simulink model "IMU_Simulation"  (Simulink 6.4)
settings: Solver=FixedStepDiscrete  StartTime=0.0  StopTime=25  FixedStep=.001  RelTol=1e-3
PreLoadFcn:
  | Script_Kalman
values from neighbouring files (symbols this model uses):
  Az = [1 -Ts ;0 1]    [Script_Kalman.m]
  Kz = 1e-3*[.4 ; -.04]    [Script_Kalman.m]
  Ts = .001    (= 0.001)    [Script_Kalman.m]
undefined symbols (not defined in the file or in its folder): dend, DiscIntNeverNeededParam, float, gaind, numd, polesd, tustin, zerosd
libraries: simulink x38
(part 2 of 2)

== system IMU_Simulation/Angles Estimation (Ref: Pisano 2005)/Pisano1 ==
  note: Probleme du filtrage de l'accelero : dephasage si variation rapide et de forte amplitude, fausse le calcul de l'offset Si on filtre moins, on se prend le biais du aux accelerations
  Gyro : Inport  Orientation=down
  Accel : Inport  Orientation=down  Port=2
  Adapt : Inport  Orientation=down  Port=3
  Constant : Constant  Orientation=left  Value=0  OutDataType=sfix(16)  OutScaling=2^0
  Gain6 : Gain  Orientation=left  Gain=1e-3  Multiplication=Matrix(K*u)  ParameterDataType=sfix(16)  ParameterScaling=2^0  OutDataType=sfix(16)  OutScaling=2^0
  Gain7 : Gain  Orientation=down  Gain=Ts  Multiplication=Matrix(K*u)  ParameterDataType=sfix(16)  ParameterScaling=2^0  OutDataType=sfix(16)  OutScaling=2^0
  Low Pass1 : Subsystem  Orientation=down  mask(DiscretizedZeroPole){Zeros=[], Poles=[-30*2*pi], Gain=30*2*pi, AbsTol=auto, SampleTime=.001, method=tustin, Wc=1}
      mask prompts: Zeros "Zeros (enter in s-main:)"; Poles "Poles (enter in s-domain:)"; Gain "Gain (enter in s-domain:)"; AbsTol "Absolute tolerance:"; SampleTime "Sample time:"; Wc "Critical Frequency (Hz):"
      mask help: Continuous mask uses c2d to transform parameters onto the Discrete Zero-Pole block inside.
      mask init:
      | st=SampleTime;
      | if length(st)>1
      |     st=SampleTime(1);
      | end
      | if(st>0)
      |     [zerosd,polesd,gaind] = sldiscutil('disczpk', {st,method,Wc,Zeros,Poles,Gain});
      | end	
      | s = get_param(gcb,'maskvalues');
      | zeross = s{1};
      | poless = s{2};
      | gainss = s{3};
      | %zerosc = eval(zeross);
      | %polesc = eval(poless);
      | %gainsc = eval(gainss);
      | sldiscutil('initzpkmask', st);
      | if(st==0)
      | set_param([gcb '/Zero Pole'], 'AbsoluteTolerance', AbsTol);
      | end
  Multiport Switch : MultiPortSwitch  Orientation=left  Inputs=2  zeroidx=on
  Sum2 : Sum  Inputs=++|  OutDataType=sfix(16)  OutScaling=2^0
  Sum4 : Sum  Inputs=++|  OutDataType=sfix(16)  OutScaling=2^0
  Sum5 : Sum  Orientation=left  Inputs=+-  OutDataType=sfix(16)  OutScaling=2^0
  Unit Delay2 : UnitDelay  SampleTime=-1
  Position : Outport  Orientation=up  OutDataType=sfix(16)  OutScaling=2^0
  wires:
  Sum4/1 -> Unit Delay2/1, Position/1
  Constant/1 -> Multiport Switch/2
  Gain6/1 -> Multiport Switch/3
  Adapt/1 -> Multiport Switch/1
  Multiport Switch/1 -> Sum4/1
  Sum2/1 -> Sum4/2
  Sum5/1 -> Gain6/1
  Gain7/1 -> Sum2/1
  Accel/1 -> Low Pass1/1(In1)
  Gyro/1 -> Gain7/1
  Unit Delay2/1 -> Sum5/2, Sum2/2
  Low Pass1/1(Out1) -> Sum5/1

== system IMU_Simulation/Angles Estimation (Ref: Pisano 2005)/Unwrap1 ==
  Estimated Angle : Inport
  Compare To Constant : simulink/Logic and Bit Operations/Compare To Constant  SystemSampleTime=-1  relop=>  const=180  LogicOutDataTypeMode=uint8  ZeroCross=off
  Compare To Constant1 : simulink/Logic and Bit Operations/Compare To Constant  SystemSampleTime=-1  relop=<  const=-180  LogicOutDataTypeMode=uint8  ZeroCross=off
  Compare To Zero : simulink/Logic and Bit Operations/Compare To Zero  SystemSampleTime=-1  relop=~=  LogicOutDataTypeMode=uint8  ZeroCross=off
  Difference : simulink/Discrete/Difference  SystemSampleTime=-1  ICPrevInput=0.0  OutDataType=sfix(16)  OutScaling=2^-10  DoSatur=off
  Discrete-Time Integrator : DiscreteIntegrator  gainval=1000  SampleTime=-1  OutDataType=sfix(16)  OutScaling=2^0  ICPrevOutput=DiscIntNeverNeededParam  ICPrevScaledInput=DiscIntNeverNeededParam
  Logical Operator : Logic  Orientation=up  Operator=NOR  AllPortsSameDT=off  OutDataTypeMode=boolean
  Lookup Table : Lookup  Orientation=left  InputValues=[-500 -195 195]  OutputValues=[+360 0 -360]  LookUpMeth=Use Input Below  OutDataType=sfix(16)  OutScaling=2^0
  Merge : Merge  Inputs=3
  Sum2 : Sum  OutDataType=sfix(16)  OutScaling=2^0
  unwrap : Subsystem  TreatAsAtomicUnit=on
  unwrap1 : Subsystem  TreatAsAtomicUnit=on
  unwrap2 : Subsystem  TreatAsAtomicUnit=on
  unwrap angle : Outport
  Wrap : Outport  Port=2
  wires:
  Discrete-Time Integrator/1 -> unwrap angle/1, Lookup Table/1
  Estimated Angle/1 -> Difference/1
  unwrap1/1(Out1) -> Merge/3
  unwrap/1(Out1) -> Merge/2
  unwrap2/1(Out1) -> Merge/1
  Logical Operator/1 -> unwrap2/Enable
  Compare To Constant1/1 -> Logical Operator/2, unwrap1/Enable
  Compare To Constant/1 -> unwrap/Enable, Logical Operator/1
  Difference/1 -> unwrap2/1(In1), unwrap1/1(In1), Compare To Constant1/1, unwrap/1(In1), Compare To Constant/1
  Sum2/1 -> Discrete-Time Integrator/1
  Merge/1 -> Sum2/2
  Lookup Table/1 -> Sum2/1, Compare To Zero/1
  Compare To Zero/1 -> Wrap/1

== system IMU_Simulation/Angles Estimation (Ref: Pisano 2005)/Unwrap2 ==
  Estimated Angle : Inport
  Compare To Constant : simulink/Logic and Bit Operations/Compare To Constant  SystemSampleTime=-1  relop=>  const=180  LogicOutDataTypeMode=uint8  ZeroCross=off
  Compare To Constant1 : simulink/Logic and Bit Operations/Compare To Constant  SystemSampleTime=-1  relop=<  const=-180  LogicOutDataTypeMode=uint8  ZeroCross=off
  Compare To Zero : simulink/Logic and Bit Operations/Compare To Zero  SystemSampleTime=-1  relop=~=  LogicOutDataTypeMode=uint8  ZeroCross=off
  Difference : simulink/Discrete/Difference  SystemSampleTime=-1  ICPrevInput=0.0  OutDataType=sfix(16)  OutScaling=2^-10  DoSatur=off
  Discrete-Time Integrator : DiscreteIntegrator  gainval=1000  SampleTime=-1  OutDataType=sfix(16)  OutScaling=2^0  ICPrevOutput=DiscIntNeverNeededParam  ICPrevScaledInput=DiscIntNeverNeededParam
  Logical Operator : Logic  Orientation=up  Operator=NOR  AllPortsSameDT=off  OutDataTypeMode=boolean
  Lookup Table : Lookup  Orientation=left  InputValues=[-500 -195 195]  OutputValues=[+360 0 -360]  LookUpMeth=Use Input Below  OutDataType=sfix(16)  OutScaling=2^0
  Merge : Merge  Inputs=3
  Sum2 : Sum  OutDataType=sfix(16)  OutScaling=2^0
  unwrap : Subsystem  TreatAsAtomicUnit=on
  unwrap1 : Subsystem  TreatAsAtomicUnit=on
  unwrap2 : Subsystem  TreatAsAtomicUnit=on
  unwrap angle : Outport
  Wrap : Outport  Port=2
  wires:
  Compare To Zero/1 -> Wrap/1
  Lookup Table/1 -> Compare To Zero/1, Sum2/1
  Merge/1 -> Sum2/2
  Sum2/1 -> Discrete-Time Integrator/1
  Difference/1 -> Compare To Constant/1, unwrap/1(In1), Compare To Constant1/1, unwrap1/1(In1), unwrap2/1(In1)
  Compare To Constant/1 -> Logical Operator/1, unwrap/Enable
  Compare To Constant1/1 -> unwrap1/Enable, Logical Operator/2
  Logical Operator/1 -> unwrap2/Enable
  unwrap2/1(Out1) -> Merge/1
  unwrap/1(Out1) -> Merge/2
  unwrap1/1(Out1) -> Merge/3
  Estimated Angle/1 -> Difference/1
  Discrete-Time Integrator/1 -> Lookup Table/1, unwrap angle/1

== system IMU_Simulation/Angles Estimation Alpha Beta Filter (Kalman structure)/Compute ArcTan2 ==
  Force 1 : Inport
  Force 2 : Inport  Port=2
  Enable : EnablePort  StatesWhenEnabling=reset
  Gain1 : Gain  Gain=180/pi  ParameterDataType=sfix(16)  ParameterScaling=2^0  OutDataTypeMode=Specify via dialog  OutDataType=float('double')
  Trigonometric Function1 : Trigonometry  Operator=atan2  OutputSignalType=real
  Degree : Outport
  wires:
  Trigonometric Function1/1 -> Gain1/1
  Gain1/1 -> Degree/1
  Force 1/1 -> Trigonometric Function1/1
  Force 2/1 -> Trigonometric Function1/2

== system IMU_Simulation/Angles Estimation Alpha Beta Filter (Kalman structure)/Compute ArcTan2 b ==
  Force 1 : Inport
  Force 2 : Inport  Port=2
  Enable : EnablePort  StatesWhenEnabling=reset
  Gain1 : Gain  Gain=180/pi  ParameterDataType=sfix(16)  ParameterScaling=2^0  OutDataTypeMode=Specify via dialog  OutDataType=float('double')
  Trigonometric Function1 : Trigonometry  Operator=atan2  OutputSignalType=real
  Degree : Outport
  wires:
  Force 2/1 -> Trigonometric Function1/2
  Force 1/1 -> Trigonometric Function1/1
  Gain1/1 -> Degree/1
  Trigonometric Function1/1 -> Gain1/1

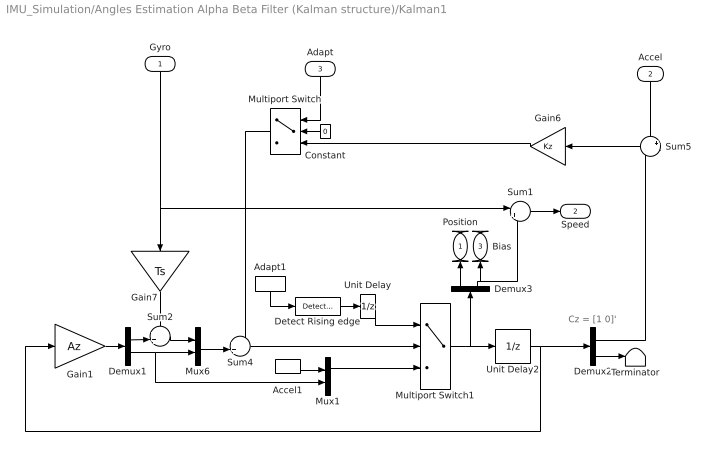
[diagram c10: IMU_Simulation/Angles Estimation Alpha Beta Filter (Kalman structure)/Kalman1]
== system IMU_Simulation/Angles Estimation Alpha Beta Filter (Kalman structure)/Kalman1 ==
  note: Cz = [1 0]'
  Gyro : Inport  Orientation=down
  Accel : Inport  Orientation=down  Port=2
  Adapt : Inport  Orientation=down  Port=3
  Accel1 : InportShadow  Port=2  LatchByCopyingInsideSignal=off
  Adapt1 : InportShadow  Orientation=down  Port=3  LatchByCopyingInsideSignal=off
  Constant : Constant  Orientation=left  Value=0  OutDataType=sfix(16)  OutScaling=2^0
  Demux1 : Demux  Outputs=2
  Demux2 : Demux  Outputs=2
  Demux3 : Demux  Orientation=up  Outputs=2
  Detect Rising edge : simulink/Logic and Bit Operations/Detect Increase  SystemSampleTime=-1  vinit=0
  Gain1 : Gain  Gain=Az  Multiplication=Matrix(K*u)  ParameterDataType=sfix(16)  ParameterScaling=2^0  OutDataType=sfix(16)  OutScaling=2^0
  Gain6 : Gain  Orientation=left  Gain=Kz  Multiplication=Matrix(K*u)  ParameterDataType=sfix(16)  ParameterScaling=2^0  OutDataType=sfix(16)  OutScaling=2^0
  Gain7 : Gain  Orientation=down  Gain=Ts  Multiplication=Matrix(K*u)  ParameterDataType=sfix(16)  ParameterScaling=2^0  OutDataType=sfix(16)  OutScaling=2^0
  Multiport Switch : MultiPortSwitch  Orientation=left  Inputs=2  zeroidx=on
  Multiport Switch1 : MultiPortSwitch  Inputs=2  zeroidx=on
  Mux1 : Mux  Inputs=2
  Mux6 : Mux  Inputs=2
  Sum1 : Sum  Inputs=|+-  OutDataType=sfix(16)  OutScaling=2^0
  Sum2 : Sum  Inputs=++|  OutDataType=sfix(16)  OutScaling=2^0
  Sum4 : Sum  Inputs=++|  OutDataType=sfix(16)  OutScaling=2^0
  Sum5 : Sum  Orientation=left  Inputs=+-  OutDataType=sfix(16)  OutScaling=2^0
  Terminator : Terminator
  Unit Delay : UnitDelay  SampleTime=-1
  Unit Delay2 : UnitDelay  SampleTime=-1
  Position : Outport  Orientation=up  OutDataType=sfix(16)  OutScaling=2^0
  Speed : Outport  Port=2  OutDataType=sfix(16)  OutScaling=2^0
  Bias : Outport  Orientation=up  Port=3  OutDataType=sfix(16)  OutScaling=2^0
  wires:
  Sum1/1 -> Speed/1
  Demux3/2 -> Sum1/2, Bias/1
  Demux3/1 -> Position/1
  Unit Delay2/1 -> Gain1/1, Demux2/1
  Unit Delay/1 -> Multiport Switch1/1
  Gyro/1 -> Sum1/1, Gain7/1
  Accel/1 -> Sum5/1
  Gain7/1 -> Sum2/1
  Sum5/1 -> Gain6/1
  Mux6/1 -> Sum4/2
  Demux1/2 -> Mux6/2, Mux1/2
  Sum2/1 -> Mux6/1
  Demux1/1 -> Sum2/2
  Gain1/1 -> Demux1/1
  Demux2/1 -> Sum5/2
  Multiport Switch/1 -> Sum4/1
  Adapt/1 -> Multiport Switch/1
  Gain6/1 -> Multiport Switch/3
  Constant/1 -> Multiport Switch/2
  Detect Rising edge/1 -> Unit Delay/1
  Multiport Switch1/1 -> Demux3/1, Unit Delay2/1
  Sum4/1 -> Multiport Switch1/2
  Adapt1/1 -> Detect Rising edge/1
  Accel1/1 -> Mux1/1
  Mux1/1 -> Multiport Switch1/3
  Demux2/2 -> Terminator/1

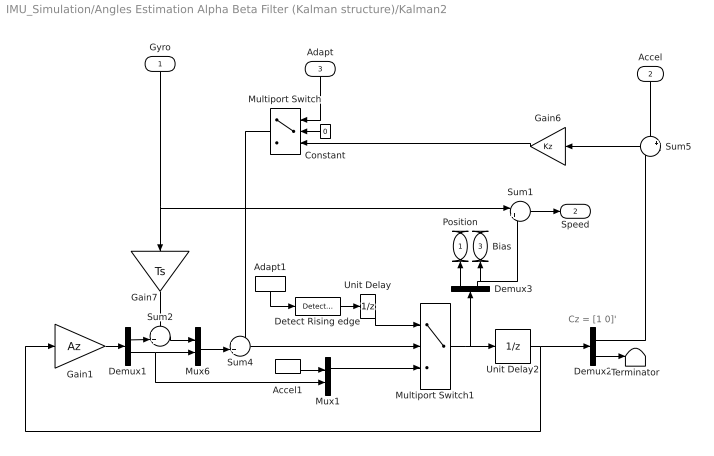
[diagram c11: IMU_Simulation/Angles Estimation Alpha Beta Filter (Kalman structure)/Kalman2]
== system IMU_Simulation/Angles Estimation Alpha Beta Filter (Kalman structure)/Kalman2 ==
  note: Cz = [1 0]'
  Gyro : Inport  Orientation=down
  Accel : Inport  Orientation=down  Port=2
  Adapt : Inport  Orientation=down  Port=3
  Accel1 : InportShadow  Port=2  LatchByCopyingInsideSignal=off
  Adapt1 : InportShadow  Orientation=down  Port=3  LatchByCopyingInsideSignal=off
  Constant : Constant  Orientation=left  Value=0  OutDataType=sfix(16)  OutScaling=2^0
  Demux1 : Demux  Outputs=2
  Demux2 : Demux  Outputs=2
  Demux3 : Demux  Orientation=up  Outputs=2
  Detect Rising edge : simulink/Logic and Bit Operations/Detect Increase  SystemSampleTime=-1  vinit=0
  Gain1 : Gain  Gain=Az  Multiplication=Matrix(K*u)  ParameterDataType=sfix(16)  ParameterScaling=2^0  OutDataType=sfix(16)  OutScaling=2^0
  Gain6 : Gain  Orientation=left  Gain=Kz  Multiplication=Matrix(K*u)  ParameterDataType=sfix(16)  ParameterScaling=2^0  OutDataType=sfix(16)  OutScaling=2^0
  Gain7 : Gain  Orientation=down  Gain=Ts  Multiplication=Matrix(K*u)  ParameterDataType=sfix(16)  ParameterScaling=2^0  OutDataType=sfix(16)  OutScaling=2^0
  Multiport Switch : MultiPortSwitch  Orientation=left  Inputs=2  zeroidx=on
  Multiport Switch1 : MultiPortSwitch  Inputs=2  zeroidx=on
  Mux1 : Mux  Inputs=2
  Mux6 : Mux  Inputs=2
  Sum1 : Sum  Inputs=|+-  OutDataType=sfix(16)  OutScaling=2^0
  Sum2 : Sum  Inputs=++|  OutDataType=sfix(16)  OutScaling=2^0
  Sum4 : Sum  Inputs=++|  OutDataType=sfix(16)  OutScaling=2^0
  Sum5 : Sum  Orientation=left  Inputs=+-  OutDataType=sfix(16)  OutScaling=2^0
  Terminator : Terminator
  Unit Delay : UnitDelay  SampleTime=-1
  Unit Delay2 : UnitDelay  SampleTime=-1
  Position : Outport  Orientation=up  OutDataType=sfix(16)  OutScaling=2^0
  Speed : Outport  Port=2  OutDataType=sfix(16)  OutScaling=2^0
  Bias : Outport  Orientation=up  Port=3  OutDataType=sfix(16)  OutScaling=2^0
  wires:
  Demux2/2 -> Terminator/1
  Mux1/1 -> Multiport Switch1/3
  Accel1/1 -> Mux1/1
  Adapt1/1 -> Detect Rising edge/1
  Sum4/1 -> Multiport Switch1/2
  Multiport Switch1/1 -> Unit Delay2/1, Demux3/1
  Detect Rising edge/1 -> Unit Delay/1
  Constant/1 -> Multiport Switch/2
  Gain6/1 -> Multiport Switch/3
  Adapt/1 -> Multiport Switch/1
  Multiport Switch/1 -> Sum4/1
  Demux2/1 -> Sum5/2
  Gain1/1 -> Demux1/1
  Demux1/1 -> Sum2/2
  Sum2/1 -> Mux6/1
  Demux1/2 -> Mux1/2, Mux6/2
  Mux6/1 -> Sum4/2
  Sum5/1 -> Gain6/1
  Gain7/1 -> Sum2/1
  Accel/1 -> Sum5/1
  Gyro/1 -> Gain7/1, Sum1/1
  Unit Delay/1 -> Multiport Switch1/1
  Unit Delay2/1 -> Demux2/1, Gain1/1
  Demux3/1 -> Position/1
  Demux3/2 -> Bias/1, Sum1/2
  Sum1/1 -> Speed/1

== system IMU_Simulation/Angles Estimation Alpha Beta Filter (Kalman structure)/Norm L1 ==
  Accel Y : Inport
  Accel Z : Inport  Port=2
  Accel X : Inport  Port=3
  Abs : Abs
  Abs1 : Abs
  Abs2 : Abs
  Sum1 : Sum  OutDataType=sfix(16)  OutScaling=2^0
  Sum3 : Sum  OutDataType=sfix(16)  OutScaling=2^0
  abs(Y)+abs(Z) : Outport
  abs(X)+abs(Z) : Outport  Port=2
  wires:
  Abs/1 -> Sum3/1
  Abs1/1 -> Sum1/1, Sum3/2
  Accel Y/1 -> Abs/1
  Accel Z/1 -> Abs1/1
  Sum3/1 -> abs(Y)+abs(Z)/1
  Abs2/1 -> Sum1/2
  Accel X/1 -> Abs2/1
  Sum1/1 -> abs(X)+abs(Z)/1

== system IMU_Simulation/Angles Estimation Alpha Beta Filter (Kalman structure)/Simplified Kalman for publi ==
  note: Cz = [1 0]'
  Gyro : Inport  Orientation=down
  Accel : Inport  Orientation=down  Port=2
  Demux1 : Demux  Outputs=2
  Demux2 : Demux  Outputs=2
  Gain1 : Gain  Gain=Az  Multiplication=Matrix(K*u)  ParameterDataType=sfix(16)  ParameterScaling=2^0  OutDataType=sfix(16)  OutScaling=2^0
  Gain6 : Gain  Orientation=left  Gain=Kz  Multiplication=Matrix(K*u)  ParameterDataType=sfix(16)  ParameterScaling=2^0  OutDataType=sfix(16)  OutScaling=2^0
  Gain7 : Gain  Orientation=down  Gain=Ts  Multiplication=Matrix(K*u)  ParameterDataType=sfix(16)  ParameterScaling=2^0  OutDataType=sfix(16)  OutScaling=2^0
  Mux6 : Mux  Inputs=2
  Sum2 : Sum  Inputs=++|  OutDataType=sfix(16)  OutScaling=2^0
  Sum4 : Sum  Inputs=++|  OutDataType=sfix(16)  OutScaling=2^0
  Sum5 : Sum  Orientation=left  Inputs=+-  OutDataType=sfix(16)  OutScaling=2^0
  Terminator : Terminator
  Unit Delay2 : UnitDelay  SampleTime=-1
  Angle Estimation : Outport  OutDataType=sfix(16)  OutScaling=2^0
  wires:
  Demux2/2 -> Terminator/1
  Sum4/1 -> Unit Delay2/1
  Demux2/1 -> Sum5/2, Angle Estimation/1
  Gain1/1 -> Demux1/1
  Demux1/1 -> Sum2/2
  Sum2/1 -> Mux6/1  "Angle Estimation"
  Demux1/2 -> Mux6/2  "Gyro Bias"
  Mux6/1 -> Sum4/2
  Sum5/1 -> Gain6/1
  Gain7/1 -> Sum2/1
  Accel/1 -> Sum5/1
  Gyro/1 -> Gain7/1
  Unit Delay2/1 -> Demux2/1, Gain1/1
  Gain6/1 -> Sum4/1

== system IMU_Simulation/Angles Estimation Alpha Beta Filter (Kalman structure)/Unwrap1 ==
  Estimated Angle : Inport
  Compare To Constant : simulink/Logic and Bit Operations/Compare To Constant  SystemSampleTime=-1  relop=>  const=180  LogicOutDataTypeMode=uint8  ZeroCross=off
  Compare To Constant1 : simulink/Logic and Bit Operations/Compare To Constant  SystemSampleTime=-1  relop=<  const=-180  LogicOutDataTypeMode=uint8  ZeroCross=off
  Compare To Zero : simulink/Logic and Bit Operations/Compare To Zero  SystemSampleTime=-1  relop=~=  LogicOutDataTypeMode=uint8  ZeroCross=off
  Difference : simulink/Discrete/Difference  SystemSampleTime=-1  ICPrevInput=0.0  OutDataType=sfix(16)  OutScaling=2^-10  DoSatur=off
  Discrete-Time Integrator : DiscreteIntegrator  gainval=1000  SampleTime=-1  OutDataType=sfix(16)  OutScaling=2^0  ICPrevOutput=DiscIntNeverNeededParam  ICPrevScaledInput=DiscIntNeverNeededParam
  Logical Operator : Logic  Orientation=up  Operator=NOR  AllPortsSameDT=off  OutDataTypeMode=boolean
  Lookup Table : Lookup  Orientation=left  InputValues=[-500 -195 195]  OutputValues=[+360 0 -360]  LookUpMeth=Use Input Below  OutDataType=sfix(16)  OutScaling=2^0
  Merge : Merge  Inputs=3
  Sum2 : Sum  OutDataType=sfix(16)  OutScaling=2^0
  unwrap : Subsystem  TreatAsAtomicUnit=on
  unwrap1 : Subsystem  TreatAsAtomicUnit=on
  unwrap2 : Subsystem  TreatAsAtomicUnit=on
  unwrap angle : Outport
  Wrap : Outport  Port=2
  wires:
  Compare To Zero/1 -> Wrap/1
  Lookup Table/1 -> Compare To Zero/1, Sum2/1
  Merge/1 -> Sum2/2
  Sum2/1 -> Discrete-Time Integrator/1
  Difference/1 -> Compare To Constant/1, unwrap/1(In1), Compare To Constant1/1, unwrap1/1(In1), unwrap2/1(In1)
  Compare To Constant/1 -> Logical Operator/1, unwrap/Enable
  Compare To Constant1/1 -> unwrap1/Enable, Logical Operator/2
  Logical Operator/1 -> unwrap2/Enable
  unwrap2/1(Out1) -> Merge/1
  unwrap/1(Out1) -> Merge/2
  unwrap1/1(Out1) -> Merge/3
  Estimated Angle/1 -> Difference/1
  Discrete-Time Integrator/1 -> Lookup Table/1, unwrap angle/1

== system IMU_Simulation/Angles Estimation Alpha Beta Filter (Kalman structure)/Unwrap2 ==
  Estimated Angle : Inport
  Compare To Constant : simulink/Logic and Bit Operations/Compare To Constant  SystemSampleTime=-1  relop=>  const=180  LogicOutDataTypeMode=uint8  ZeroCross=off
  Compare To Constant1 : simulink/Logic and Bit Operations/Compare To Constant  SystemSampleTime=-1  relop=<  const=-180  LogicOutDataTypeMode=uint8  ZeroCross=off
  Compare To Zero : simulink/Logic and Bit Operations/Compare To Zero  SystemSampleTime=-1  relop=~=  LogicOutDataTypeMode=uint8  ZeroCross=off
  Difference : simulink/Discrete/Difference  SystemSampleTime=-1  ICPrevInput=0.0  OutDataType=sfix(16)  OutScaling=2^-10  DoSatur=off
  Discrete-Time Integrator : DiscreteIntegrator  gainval=1000  SampleTime=-1  OutDataType=sfix(16)  OutScaling=2^0  ICPrevOutput=DiscIntNeverNeededParam  ICPrevScaledInput=DiscIntNeverNeededParam
  Logical Operator : Logic  Orientation=up  Operator=NOR  AllPortsSameDT=off  OutDataTypeMode=boolean
  Lookup Table : Lookup  Orientation=left  InputValues=[-500 -195 195]  OutputValues=[+360 0 -360]  LookUpMeth=Use Input Below  OutDataType=sfix(16)  OutScaling=2^0
  Merge : Merge  Inputs=3
  Sum2 : Sum  OutDataType=sfix(16)  OutScaling=2^0
  unwrap : Subsystem  TreatAsAtomicUnit=on
  unwrap1 : Subsystem  TreatAsAtomicUnit=on
  unwrap2 : Subsystem  TreatAsAtomicUnit=on
  unwrap angle : Outport
  Wrap : Outport  Port=2
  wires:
  Discrete-Time Integrator/1 -> unwrap angle/1, Lookup Table/1
  Estimated Angle/1 -> Difference/1
  unwrap1/1(Out1) -> Merge/3
  unwrap/1(Out1) -> Merge/2
  unwrap2/1(Out1) -> Merge/1
  Logical Operator/1 -> unwrap2/Enable
  Compare To Constant1/1 -> Logical Operator/2, unwrap1/Enable
  Compare To Constant/1 -> unwrap/Enable, Logical Operator/1
  Difference/1 -> unwrap2/1(In1), unwrap1/1(In1), Compare To Constant1/1, unwrap/1(In1), Compare To Constant/1
  Sum2/1 -> Discrete-Time Integrator/1
  Merge/1 -> Sum2/2
  Lookup Table/1 -> Sum2/1, Compare To Zero/1
  Compare To Zero/1 -> Wrap/1

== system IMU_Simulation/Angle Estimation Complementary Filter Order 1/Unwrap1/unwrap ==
  In1 : Inport  OutDataType=sfix(16)  OutScaling=2^0
  Enable : EnablePort
  Bias2 : Constant  Value=-360  OutDataType=sfix(16)  OutScaling=2^0
  Sum2 : Sum  OutDataType=sfix(16)  OutScaling=2^0
  Out1 : Outport  OutDataType=sfix(16)  OutScaling=2^0
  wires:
  Bias2/1 -> Sum2/2
  Sum2/1 -> Out1/1
  In1/1 -> Sum2/1

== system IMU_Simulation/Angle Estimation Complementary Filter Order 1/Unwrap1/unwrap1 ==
  In1 : Inport  OutDataType=sfix(16)  OutScaling=2^0
  Enable : EnablePort
  Bias2 : Constant  Value=360  OutDataType=sfix(16)  OutScaling=2^0
  Sum2 : Sum  OutDataType=sfix(16)  OutScaling=2^0
  Out1 : Outport  OutDataType=sfix(16)  OutScaling=2^0
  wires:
  Sum2/1 -> Out1/1
  Bias2/1 -> Sum2/2
  In1/1 -> Sum2/1

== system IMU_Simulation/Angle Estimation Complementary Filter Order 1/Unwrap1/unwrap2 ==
  In1 : Inport  OutDataType=sfix(16)  OutScaling=2^0
  Enable : EnablePort
  Out1 : Outport  OutDataType=sfix(16)  OutScaling=2^0
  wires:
  In1/1 -> Out1/1

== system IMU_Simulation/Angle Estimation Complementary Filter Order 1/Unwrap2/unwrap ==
  In1 : Inport  OutDataType=sfix(16)  OutScaling=2^0
  Enable : EnablePort
  Bias2 : Constant  Value=-360  OutDataType=sfix(16)  OutScaling=2^0
  Sum2 : Sum  OutDataType=sfix(16)  OutScaling=2^0
  Out1 : Outport  OutDataType=sfix(16)  OutScaling=2^0
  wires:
  In1/1 -> Sum2/1
  Sum2/1 -> Out1/1
  Bias2/1 -> Sum2/2

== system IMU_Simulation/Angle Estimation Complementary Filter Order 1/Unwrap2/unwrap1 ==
  In1 : Inport  OutDataType=sfix(16)  OutScaling=2^0
  Enable : EnablePort
  Bias2 : Constant  Value=360  OutDataType=sfix(16)  OutScaling=2^0
  Sum2 : Sum  OutDataType=sfix(16)  OutScaling=2^0
  Out1 : Outport  OutDataType=sfix(16)  OutScaling=2^0
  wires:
  In1/1 -> Sum2/1
  Bias2/1 -> Sum2/2
  Sum2/1 -> Out1/1

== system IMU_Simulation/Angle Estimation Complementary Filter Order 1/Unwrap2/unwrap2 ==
  In1 : Inport  OutDataType=sfix(16)  OutScaling=2^0
  Enable : EnablePort
  Out1 : Outport  OutDataType=sfix(16)  OutScaling=2^0
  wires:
  In1/1 -> Out1/1

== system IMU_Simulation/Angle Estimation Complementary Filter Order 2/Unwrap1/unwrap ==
  In1 : Inport  OutDataType=sfix(16)  OutScaling=2^0
  Enable : EnablePort
  Bias2 : Constant  Value=-360  OutDataType=sfix(16)  OutScaling=2^0
  Sum2 : Sum  OutDataType=sfix(16)  OutScaling=2^0
  Out1 : Outport  OutDataType=sfix(16)  OutScaling=2^0
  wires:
  In1/1 -> Sum2/1
  Sum2/1 -> Out1/1
  Bias2/1 -> Sum2/2

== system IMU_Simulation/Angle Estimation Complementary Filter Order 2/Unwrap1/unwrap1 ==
  In1 : Inport  OutDataType=sfix(16)  OutScaling=2^0
  Enable : EnablePort
  Bias2 : Constant  Value=360  OutDataType=sfix(16)  OutScaling=2^0
  Sum2 : Sum  OutDataType=sfix(16)  OutScaling=2^0
  Out1 : Outport  OutDataType=sfix(16)  OutScaling=2^0
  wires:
  In1/1 -> Sum2/1
  Bias2/1 -> Sum2/2
  Sum2/1 -> Out1/1

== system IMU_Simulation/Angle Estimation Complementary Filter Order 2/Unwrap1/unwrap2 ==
  In1 : Inport  OutDataType=sfix(16)  OutScaling=2^0
  Enable : EnablePort
  Out1 : Outport  OutDataType=sfix(16)  OutScaling=2^0
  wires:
  In1/1 -> Out1/1

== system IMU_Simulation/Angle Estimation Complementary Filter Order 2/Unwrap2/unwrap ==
  In1 : Inport  OutDataType=sfix(16)  OutScaling=2^0
  Enable : EnablePort
  Bias2 : Constant  Value=-360  OutDataType=sfix(16)  OutScaling=2^0
  Sum2 : Sum  OutDataType=sfix(16)  OutScaling=2^0
  Out1 : Outport  OutDataType=sfix(16)  OutScaling=2^0
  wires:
  Bias2/1 -> Sum2/2
  Sum2/1 -> Out1/1
  In1/1 -> Sum2/1

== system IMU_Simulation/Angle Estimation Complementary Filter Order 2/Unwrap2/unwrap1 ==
  In1 : Inport  OutDataType=sfix(16)  OutScaling=2^0
  Enable : EnablePort
  Bias2 : Constant  Value=360  OutDataType=sfix(16)  OutScaling=2^0
  Sum2 : Sum  OutDataType=sfix(16)  OutScaling=2^0
  Out1 : Outport  OutDataType=sfix(16)  OutScaling=2^0
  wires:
  Sum2/1 -> Out1/1
  Bias2/1 -> Sum2/2
  In1/1 -> Sum2/1

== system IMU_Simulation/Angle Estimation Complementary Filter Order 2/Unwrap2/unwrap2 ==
  In1 : Inport  OutDataType=sfix(16)  OutScaling=2^0
  Enable : EnablePort
  Out1 : Outport  OutDataType=sfix(16)  OutScaling=2^0
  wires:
  In1/1 -> Out1/1

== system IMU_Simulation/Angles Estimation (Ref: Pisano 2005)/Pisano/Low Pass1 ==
  In1 : Inport  OutDataType=sfix(16)  OutScaling=2^0
  Discrete Zero-Pole : DiscreteZeroPole  Zeros=zerosd  Poles=polesd  Gain=gaind  SampleTime=SampleTime
  Out1 : Outport  OutDataType=sfix(16)  OutScaling=2^0
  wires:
  Discrete Zero-Pole/1 -> Out1/1
  In1/1 -> Discrete Zero-Pole/1

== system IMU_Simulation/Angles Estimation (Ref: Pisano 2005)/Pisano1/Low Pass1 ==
  In1 : Inport  OutDataType=sfix(16)  OutScaling=2^0
  Discrete Zero-Pole : DiscreteZeroPole  Zeros=zerosd  Poles=polesd  Gain=gaind  SampleTime=SampleTime
  Out1 : Outport  OutDataType=sfix(16)  OutScaling=2^0
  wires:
  In1/1 -> Discrete Zero-Pole/1
  Discrete Zero-Pole/1 -> Out1/1

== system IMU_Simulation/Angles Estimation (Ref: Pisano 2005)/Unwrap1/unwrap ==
  In1 : Inport  OutDataType=sfix(16)  OutScaling=2^0
  Enable : EnablePort
  Bias2 : Constant  Value=-360  OutDataType=sfix(16)  OutScaling=2^0
  Sum2 : Sum  OutDataType=sfix(16)  OutScaling=2^0
  Out1 : Outport  OutDataType=sfix(16)  OutScaling=2^0
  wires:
  Bias2/1 -> Sum2/2
  Sum2/1 -> Out1/1
  In1/1 -> Sum2/1

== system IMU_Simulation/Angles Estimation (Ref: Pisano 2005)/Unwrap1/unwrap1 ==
  In1 : Inport  OutDataType=sfix(16)  OutScaling=2^0
  Enable : EnablePort
  Bias2 : Constant  Value=360  OutDataType=sfix(16)  OutScaling=2^0
  Sum2 : Sum  OutDataType=sfix(16)  OutScaling=2^0
  Out1 : Outport  OutDataType=sfix(16)  OutScaling=2^0
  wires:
  Sum2/1 -> Out1/1
  Bias2/1 -> Sum2/2
  In1/1 -> Sum2/1

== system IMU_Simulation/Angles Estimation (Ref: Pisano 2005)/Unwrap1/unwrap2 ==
  In1 : Inport  OutDataType=sfix(16)  OutScaling=2^0
  Enable : EnablePort
  Out1 : Outport  OutDataType=sfix(16)  OutScaling=2^0
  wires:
  In1/1 -> Out1/1

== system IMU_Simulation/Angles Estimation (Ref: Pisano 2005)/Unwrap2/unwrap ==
  In1 : Inport  OutDataType=sfix(16)  OutScaling=2^0
  Enable : EnablePort
  Bias2 : Constant  Value=-360  OutDataType=sfix(16)  OutScaling=2^0
  Sum2 : Sum  OutDataType=sfix(16)  OutScaling=2^0
  Out1 : Outport  OutDataType=sfix(16)  OutScaling=2^0
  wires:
  In1/1 -> Sum2/1
  Sum2/1 -> Out1/1
  Bias2/1 -> Sum2/2

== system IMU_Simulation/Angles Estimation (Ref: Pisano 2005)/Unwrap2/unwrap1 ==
  In1 : Inport  OutDataType=sfix(16)  OutScaling=2^0
  Enable : EnablePort
  Bias2 : Constant  Value=360  OutDataType=sfix(16)  OutScaling=2^0
  Sum2 : Sum  OutDataType=sfix(16)  OutScaling=2^0
  Out1 : Outport  OutDataType=sfix(16)  OutScaling=2^0
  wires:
  In1/1 -> Sum2/1
  Bias2/1 -> Sum2/2
  Sum2/1 -> Out1/1

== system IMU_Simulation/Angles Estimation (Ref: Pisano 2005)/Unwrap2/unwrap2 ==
  In1 : Inport  OutDataType=sfix(16)  OutScaling=2^0
  Enable : EnablePort
  Out1 : Outport  OutDataType=sfix(16)  OutScaling=2^0
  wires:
  In1/1 -> Out1/1

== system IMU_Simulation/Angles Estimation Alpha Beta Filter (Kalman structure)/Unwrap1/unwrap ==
  In1 : Inport  OutDataType=sfix(16)  OutScaling=2^0
  Enable : EnablePort
  Bias2 : Constant  Value=-360  OutDataType=sfix(16)  OutScaling=2^0
  Sum2 : Sum  OutDataType=sfix(16)  OutScaling=2^0
  Out1 : Outport  OutDataType=sfix(16)  OutScaling=2^0
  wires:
  In1/1 -> Sum2/1
  Sum2/1 -> Out1/1
  Bias2/1 -> Sum2/2

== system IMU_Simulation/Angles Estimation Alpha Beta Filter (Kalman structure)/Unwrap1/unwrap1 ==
  In1 : Inport  OutDataType=sfix(16)  OutScaling=2^0
  Enable : EnablePort
  Bias2 : Constant  Value=360  OutDataType=sfix(16)  OutScaling=2^0
  Sum2 : Sum  OutDataType=sfix(16)  OutScaling=2^0
  Out1 : Outport  OutDataType=sfix(16)  OutScaling=2^0
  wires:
  In1/1 -> Sum2/1
  Bias2/1 -> Sum2/2
  Sum2/1 -> Out1/1

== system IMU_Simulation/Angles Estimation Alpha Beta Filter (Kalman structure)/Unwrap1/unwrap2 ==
  In1 : Inport  OutDataType=sfix(16)  OutScaling=2^0
  Enable : EnablePort
  Out1 : Outport  OutDataType=sfix(16)  OutScaling=2^0
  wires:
  In1/1 -> Out1/1

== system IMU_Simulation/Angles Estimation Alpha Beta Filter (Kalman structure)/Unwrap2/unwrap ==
  In1 : Inport  OutDataType=sfix(16)  OutScaling=2^0
  Enable : EnablePort
  Bias2 : Constant  Value=-360  OutDataType=sfix(16)  OutScaling=2^0
  Sum2 : Sum  OutDataType=sfix(16)  OutScaling=2^0
  Out1 : Outport  OutDataType=sfix(16)  OutScaling=2^0
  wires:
  Bias2/1 -> Sum2/2
  Sum2/1 -> Out1/1
  In1/1 -> Sum2/1

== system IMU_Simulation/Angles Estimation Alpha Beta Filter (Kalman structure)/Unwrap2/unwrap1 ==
  In1 : Inport  OutDataType=sfix(16)  OutScaling=2^0
  Enable : EnablePort
  Bias2 : Constant  Value=360  OutDataType=sfix(16)  OutScaling=2^0
  Sum2 : Sum  OutDataType=sfix(16)  OutScaling=2^0
  Out1 : Outport  OutDataType=sfix(16)  OutScaling=2^0
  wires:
  Sum2/1 -> Out1/1
  Bias2/1 -> Sum2/2
  In1/1 -> Sum2/1

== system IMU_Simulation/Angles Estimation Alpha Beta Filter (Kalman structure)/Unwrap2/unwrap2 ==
  In1 : Inport  OutDataType=sfix(16)  OutScaling=2^0
  Enable : EnablePort
  Out1 : Outport  OutDataType=sfix(16)  OutScaling=2^0
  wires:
  In1/1 -> Out1/1
